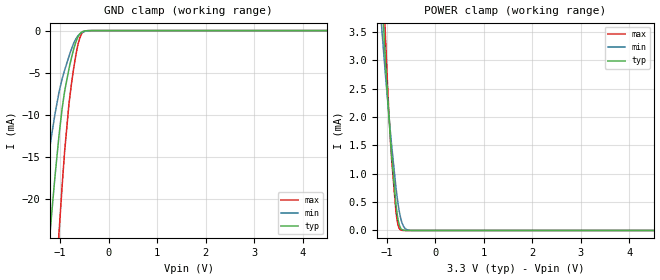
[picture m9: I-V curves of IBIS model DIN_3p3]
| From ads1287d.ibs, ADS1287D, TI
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|   Model
[Model]   DIN_3p3
Model_type   Input
Vinl = 0.99
Vinh = 2.31
|   typ   min   max
C_comp   2.259pF   1.924pF   2.539pF
[Voltage Range]   3.3   3   3.6
[Temperature Range]   27   125   -40
[Power Clamp Reference]   3.3   3   3.6
[GND Clamp Reference]   0   0   0
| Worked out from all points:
|   GND clamp passes 1 mA (typ) near -0.65 V on its own axis
|   POWER clamp passes 1 mA (typ) near -0.87 V on its own axis
[GND Clamp]
|   Voltage   I(typ)   I(min)   I(max)
-3.3V     -211.9mA   -145.2mA   -269mA
-1.459V   -43.27mA   -25.18mA   -68.11mA
-1.36V    -35.47mA   -20.42mA   -57.65mA
-1.201V   -23.84mA   -13.58mA   -41.37mA
-1.023V   -12.64mA   -7.415mA   -24.28mA
-1.013V   -12.1mA    -7.14mA    -23.39mA
-904.2mV  -7.219mA   -4.697mA   -14.35mA
-795.3mV  -4.033mA   -2.729mA   -7.768mA
-656.7mV  -1.121mA   -845.9uA   -2.418mA
-597.3mV  -437.7uA   -436.7uA   -982.7uA
-528mV    -100uA     -179.1uA   -203.9uA
6.6V      0A         0A         0A
[POWER Clamp]
|   Voltage   I(typ)   I(min)   I(max)
-3.3V     49.01mA    38.75mA    59.65mA
-1.102V   4.165mA    3.532mA    4.992mA
-1.043V   3.199mA    2.887mA    3.703mA
-1.033V   3.048mA    2.784mA    3.497mA
-963.6mV  2.082mA    2.086mA    2.174mA
-904.2mV  1.36mA     1.524mA    1.281mA
-795.3mV  338.6uA    636.6uA    218.2uA
-755.7mV  136uA      395.9uA    56.96uA
-706.2mV  29.13uA    187.3uA    6.642uA
-627mV    1.706uA    38.45uA    186.2nA
-488.4mV  0A         918nA      0A
6.6V      0A         0A         0A
